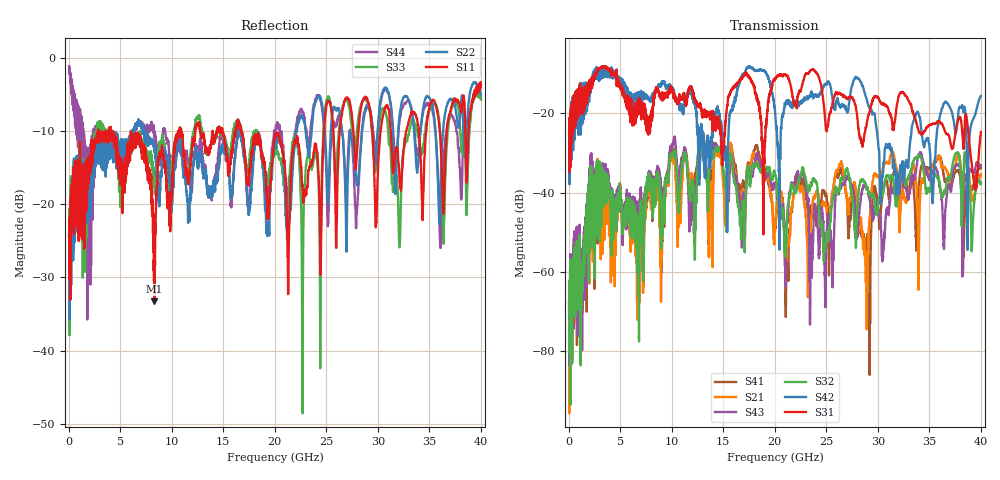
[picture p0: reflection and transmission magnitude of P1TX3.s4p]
!Agilent Technologies,N5245A,MY49151084,A.09.20.08
!Agilent N5245A: A.09.20.08
!Date: Thursday, March 01, 2012 13:23:42
!Correction: S11(Full 4 Port(1,2,3,4))
!S12(Full 4 Port(1,2,3,4))
!S13(Full 4 Port(1,2,3,4))
!S14(Full 4 Port(1,2,3,4))
!S21(Full 4 Port(1,2,3,4))
!S22(Full 4 Port(1,2,3,4))
!S23(Full 4 Port(1,2,3,4))
!S24(Full 4 Port(1,2,3,4))
!S31(Full 4 Port(1,2,3,4))
!S32(Full 4 Port(1,2,3,4))
!S33(Full 4 Port(1,2,3,4))
!S34(Full 4 Port(1,2,3,4))
!S41(Full 4 Port(1,2,3,4))
!S42(Full 4 Port(1,2,3,4))
!S43(Full 4 Port(1,2,3,4))
!S44(Full 4 Port(1,2,3,4))
!S4P File: Measurements: <S11,S12,S13,S14>,
!<S21,S22,S23,S24>,
!<S31,S32,S33,S34>,
!<S41,S42,S43,S44>:
# Hz S  dB  R 50
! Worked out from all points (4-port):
!   3996 points, 50 MHz to 40 GHz, reference 50 ohm
!   strongest paths, dB at 50 MHz, 10.04 GHz, 20.03 GHz, 30.02 GHz, 40 GHz:
!     S31: -25.3, -14.0, -11.4, -16.2, -24.7
!     S42: -24.8, -13.6, -19.7, -27.1, -15.6
!     S32: -67.4, -30.3, -35.4, -43.3, -37.5
!     S43: -68.3, -28.1, -38.1, -44.4, -33.1
!     S21: -64.6, -31.2, -49.1, -36.0, -35.6
!     S41: -67.5, -29.5, -49.4, -44.1, -33.6
!   lowest |S11| = -33.3 dB at 8.31 GHz (marker M1), VSWR 1.04, Z = 52 - j0.859 ohm
!   |S11| at or under -10 dB: start of sweep to 2.878 GHz; 4.111 GHz to 10.7 GHz (6.587 GHz wide, 89 % of centre); 16.75 GHz to 24.77 GHz (8.021 GHz wide, 38.6 % of centre)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
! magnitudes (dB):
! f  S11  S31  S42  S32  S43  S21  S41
! 50 MHz  -24.3  -25.3  -24.8  -67.4  -68.3  -64.6  -67.5
! 2.18 GHz  -14.0  -12.5  -13.4  -33.3  -30.1  -33.4  -30.1
! 8.31 GHz  -33.3  -16.2  -15.1  -39.3  -37.5  -39.1  -38.5
! 26.41 GHz  -8.7  -15.3  -18.3  -36.5  -38.8  -32.4  -34.0
! 28.88 GHz  -5.4  -23.5  -16.1  -38.4  -38.4  -59.0  -52.7
! 31.36 GHz  -12.7  -21.7  -29.5  -35.8  -38.9  -29.9  -36.4
! 40 GHz  -4.1  -24.7  -15.6  -37.5  -33.1  -35.6  -33.6
